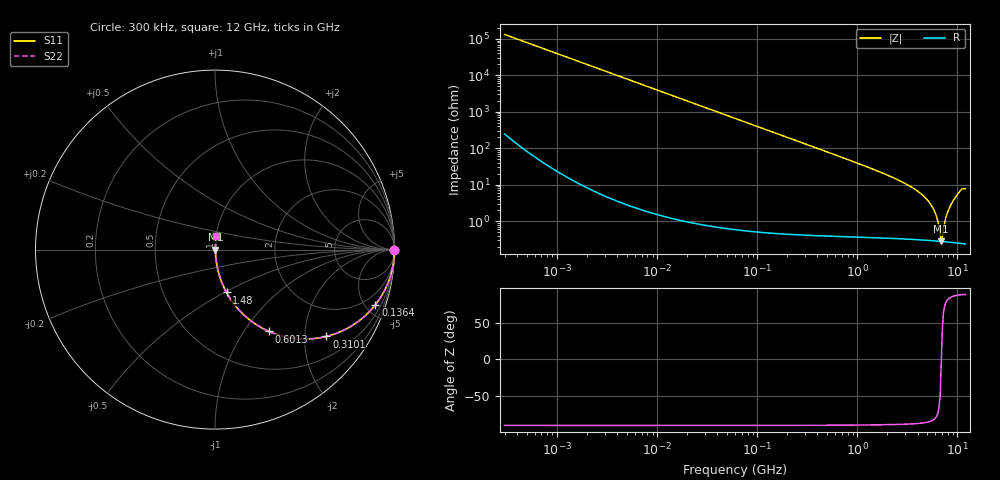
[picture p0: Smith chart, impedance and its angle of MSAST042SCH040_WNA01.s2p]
! MSAST042SCH040_WNA01  S-PARAMETER MODEL  ( General Type )
! Model Generated by TAIYO YUDEN Corporation (http://www.ty-top.com)
! Version 1.0
! TAIYO YUDEN Control No. 150820
! Copyright(c) 2015 TAIYO YUDEN CO.,LTD. All Rights Reserved.
! Product Description (link to TY-COMPAS)
! https://ds.yuden.co.jp/TYCOMPAS/or/detail?pn=MSAST042SCH040BWNA01&u=M
! Products Name : Multilayer Ceramic Capacitors
! Characteristics :
!  Capacitance : 4 pF , Rated Voltage : 25V , TCC : CH / C0H
!  Case Size : 0.4 x 0.2 / 0.016 x 0.008 [mm/inch] , Thickness : 0.2 / 0.008 [mm/inch]
!  (Conditions: Temperature = 25 degC , DC Bias Current/Voltage = 0A / 0V)
! External Node Assignments :
!  1  o---| |---o  2
! GND o---------o GND
! Frequency Range : 0.3MHz  -  12000MHz  [ 401 STEP ]
# MHz S RI R 50
! Freq[MHz].  S11 Real  S11 Imag  S21 Real  S21 Imag  S12 Real  S12 Imag  S22 Real  S22 Imag
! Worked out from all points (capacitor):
!   401 points, 300 kHz to 12 GHz, reference 50 ohm
!   read as one part in series: C = 4 pF near 316.3 kHz
!   lowest |Z| = 278 mohm at 6.88 GHz (marker M1)
!   series resonance near 6.904 GHz, so ESL is about 130 pH
!   S11 on the Smith chart (normalised r, x): 300 kHz: open; 136.4 MHz: 1.01, -5.83; 310.1 MHz: 1.01, -2.56; 601.3 MHz: 1.01, -1.31; 1.48 GHz: 1.01, -0.51; 12 GHz: 1.00, +0.15
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0.3  1 -0.000755  1.96e-06 0.000755  1.96e-06 0.000755  1 -0.000755
1.769972  1 -0.00445  2.17e-05 0.00445  2.17e-05 0.00445  1 -0.00445
10.44266  0.9993 -0.0263  0.0007 0.0263  0.0007 0.0263  0.9993 -0.0263
60  0.9776 -0.1475  0.0224 0.1475  0.0224 0.1475  0.9776 -0.1475
136.3989  0.8942 -0.3068  0.1058 0.3068  0.1058 0.3068  0.8942 -0.3068
310.0777  0.6204 -0.4837  0.3796 0.4837  0.3796 0.4837  0.6204 -0.4837
353.9943  0.5562 -0.495  0.4438 0.495  0.4438 0.495  0.5562 -0.495
601.3112  0.302 -0.4562  0.698 0.4562  0.698 0.4562  0.302 -0.4562
918.7169  0.1552 -0.3578  0.8448 0.3578  0.8448 0.3578  0.1552 -0.3578
1480.043  0.0645 -0.2389  0.9355 0.2389  0.9355 0.2389  0.0645 -0.2389
2088.533  0.0321 -0.1668  0.9679 0.1668  0.9679 0.1668  0.0321 -0.1668
3547.679  0.00983 -0.0815  0.9902 0.0815  0.9902 0.0815  0.00983 -0.0815
4875.354  0.00462 -0.0407  0.9954 0.0407  0.9954 0.0407  0.00462 -0.0407
5868.704  0.0032 -0.0188  0.9968 0.0188  0.9968 0.0188  0.0032 -0.0188
6188.031  0.00298 -0.0127  0.997 0.0127  0.997 0.0127  0.00298 -0.0127
6699.894  0.00278 -0.00357  0.9972 0.00357  0.9972 0.00357  0.00278 -0.00357
6879.757  0.00275 -0.000372  0.9973 0.000372  0.9973 0.000372  0.00275 -0.000372
7254.098  0.00274 0.00565  0.9973 -0.00565  0.9973 -0.00565  0.00274 0.00565
7854.144  0.00289 0.0152  0.9971 -0.0152  0.9971 -0.0152  0.00289 0.0152
8732.115  0.00349 0.03  0.9965 -0.03  0.9965 -0.03  0.00349 0.03
10511.28  0.00661 0.0642  0.9934 -0.0642  0.9934 -0.0642  0.00661 0.0642
12000  0.00821 0.0762  0.9918 -0.0762  0.9918 -0.0762  0.00821 0.0762
